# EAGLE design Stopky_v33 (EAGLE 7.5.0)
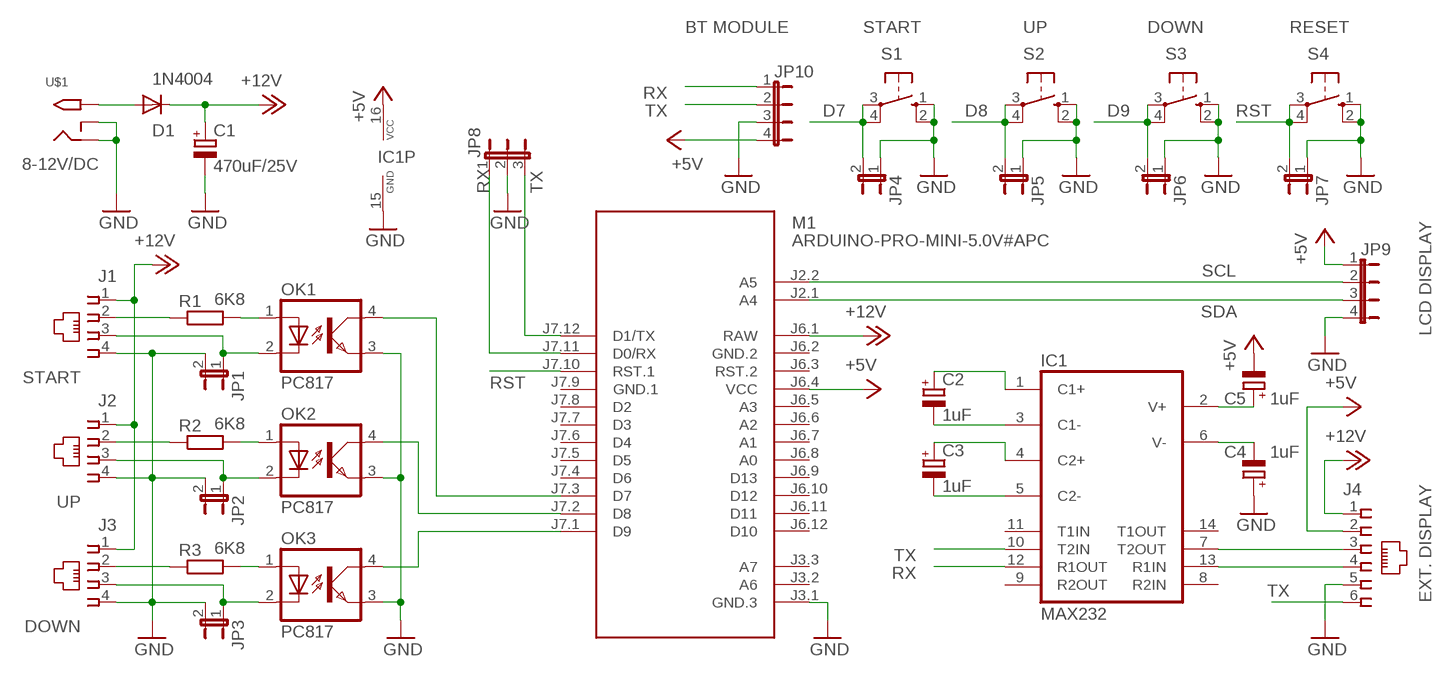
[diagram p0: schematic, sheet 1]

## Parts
C1  470uF/25V  CPOL-EUE3.5-8  [E3,5-8]
C2  1uF  CPOL-EUE2-5  [E2-5]
C3  1uF  CPOL-EUE2-5  [E2-5]
C4  1uF  CPOL-EUE2-5  [E2-5]
C5  1uF  CPOL-EUE2-5  [E2-5]
D1  1N4004  [DO41-10]
IC1  MAX232  [DIL16]
J1  215875-3  [215875-3]
J2  215875-3  [215875-3]
J3  215875-3  [215875-3]
J4  520250-3  [520250-3]
JP1  JP1E  [JP1]
JP2  JP1E  [JP1]
JP3  JP1E  [JP1]
JP4  JP1E  [JP1]
JP5  JP1E  [JP1]
JP6  JP1E  [JP1]
JP7  JP1E  [JP1]
JP8  JP2E  [JP2]
JP9  JP4E  [JP4]
JP10  JP4E  [JP4]
M1  ARDUINO-PRO-MINI-5.0V#APC  [ARDUINO-PRO-MINI#APC]
OK1  PC817  [DIL04]
OK2  PC817  [DIL04]
OK3  PC817  [DIL04]
R1  6K8  R-EU_0207/10  [0207/10]
R2  6K8  R-EU_0207/10  [0207/10]
R3  6K8  R-EU_0207/10  [0207/10]
S1  10-XX  [B3F-10XX]
S2  10-XX  [B3F-10XX]
S3  10-XX  [B3F-10XX]
S4  10-XX  [B3F-10XX]
U$1  2.1MMJACKTHM  [PJ-102A]

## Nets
+5V: C5.- IC1.16(VCC) J4.2 JP9.1 JP10.4 M1.J6.4(VCC)
+12V: C1.+ D1.C J1.1 J2.1 J3.1 J4.1 M1.J6.1(RAW)
D7: JP4.2 M1.J7.3(D7) OK1.4(COL) S1.3(P) S1.4(P1)
D8: JP5.2 M1.J7.2(D8) OK2.4(COL) S2.3(P) S2.4(P1)
D9: JP6.2 M1.J7.1(D9) OK3.4(COL) S3.3(P) S3.4(P1)
GND: C1.- C4.+ IC1.15(GND) J1.4 J2.4 J3.4 J4.5 JP1.2 JP2.2 JP3.2 JP4.1 JP5.1 JP6.1 JP7.1 JP8.2 JP9.4 JP10.3 M1.J3.1(GND.3) OK1.3(EMIT) OK2.3(EMIT) OK3.3(EMIT) S1.1(S) S1.2(S1) S2.1(S) S2.2(S1) S3.1(S) S3.2(S1) S4.1(S) S4.2(S1) U$1.RING U$1.RING_SW
N$1: D1.A U$1.TIP
N$2: J3.2 R3.1
N$3: J2.2 R2.1
N$4: J1.2 R1.1
N$5: OK1.1(A) R1.2
N$6: OK2.1(A) R2.2
N$7: OK3.1(A) R3.2
N$8: C2.+ IC1.1(C1+)
N$9: J1.3 JP1.1 OK1.2(C)
N$10: J2.3 JP2.1 OK2.2(C)
N$11: J3.3 JP3.1 OK3.2(C)
N$15: C2.- IC1.3(C1-)
N$16: C3.+ IC1.4(C2+)
N$17: C3.- IC1.5(C2-)
N$18: C4.- IC1.6(V-)
N$19: C5.+ IC1.2(V+)
N$20: IC1.7(T2OUT) J4.3
N$21: IC1.13(R1IN) J4.4
RST: JP7.2 M1.J7.10(RST.1) S4.3(P) S4.4(P1)
RX: IC1.12(R1OUT) JP8.1 JP10.1 M1.J7.11(D0/RX)
SCL: JP9.2 M1.J2.2(A5)
SDA: JP9.3 M1.J2.1(A4)
TX: IC1.10(T2IN) J4.6 JP8.3 JP10.2 M1.J7.12(D1/TX)
Unconnected: IC1.8(R2IN) IC1.9(R2OUT) IC1.11(T1IN) IC1.14(T1OUT) M1.J3.2(A6) M1.J3.3(A7) M1.J6.3(RST.2) M1.J6.5(A3) M1.J6.6(A2) M1.J6.7(A1) M1.J6.8(A0) M1.J6.9(D13) M1.J6.10(D12) M1.J6.11(D11) M1.J6.12(D10) M1.J7.4(D6) M1.J7.5(D5) M1.J7.6(D4) M1.J7.7(D3) M1.J7.8(D2)

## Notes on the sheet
- BT MODULE | START | UP | DOWN | RESET
- RX
- TX | D7 | D8 | D9 | RST
- 8-12V/DC
- RX | TX
- SCL
- SDA
- LCD DISPLAY
- START
- RST
- UP
- TX
- RX
- TX
- EXT. DISPLAY
- DOWN

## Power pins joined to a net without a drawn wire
GND.1: M1.J7.9(GND.1)
GND.2: M1.J6.2(GND.2)

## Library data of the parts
C1-C5 = rcl:CPOL-EU: POLARIZED CAPACITOR, European symbol
D1 = diode:1N4004: DIODE
IC1 = maxim:MAX232: RS232 TRANSCEIVER; MF: MAXIM; MPN: MAX232ACPE+; OC_FARNELL: 9723773; OC_NEWARK: 68K4544
J1-J3 = con-amp:215875-3: AMP connector
J4 = con-amp:520250-3: AMP connector
JP1-JP7 = jumper:JP1E: JUMPER
JP8 = jumper:JP2E: JUMPER
JP9 JP10 = jumper:JP4E: JUMPER
M1 = Arduino-module:ARDUINO-PRO-MINI-*#APC: Arduino Pro Mini with angle programming connector
OK1-OK3 = optocoupler:PC817: SHARP OPTO COUPLER; MPN: PC817X4J000F; OC_FARNELL: 9707727; OC_NEWARK: 97K7059
R1-R3 = rcl:R-EU_: RESISTOR, European symbol
S1-S4 = switch-omron:10-XX: OMRON SWITCH; MPN: B3F-1000; OC_FARNELL: 176432; OC_NEWARK: 36M3542
U$1 = adafruit:2.1MMJACK: 2.1mm x 5.5mm THM DC jack with internal switch. Digikey part #PJ-102A, 4UCON part #05537 2.1mm x 5.5mm SMT DC jack with internal switch. Digikey part #PJ-002A-SMT, 4UCON part #03267 By microbuilder.eu & adafruit.com

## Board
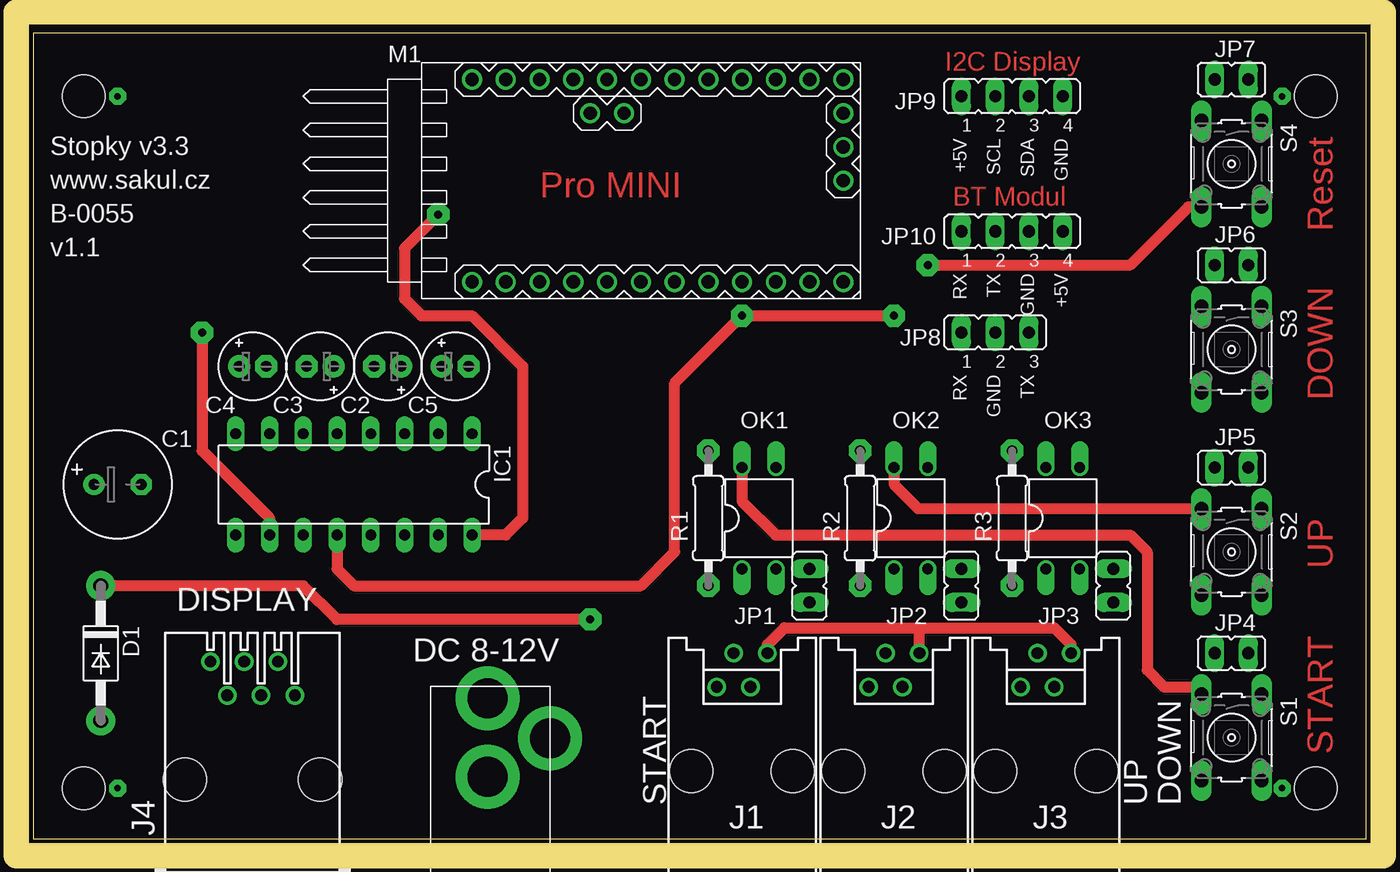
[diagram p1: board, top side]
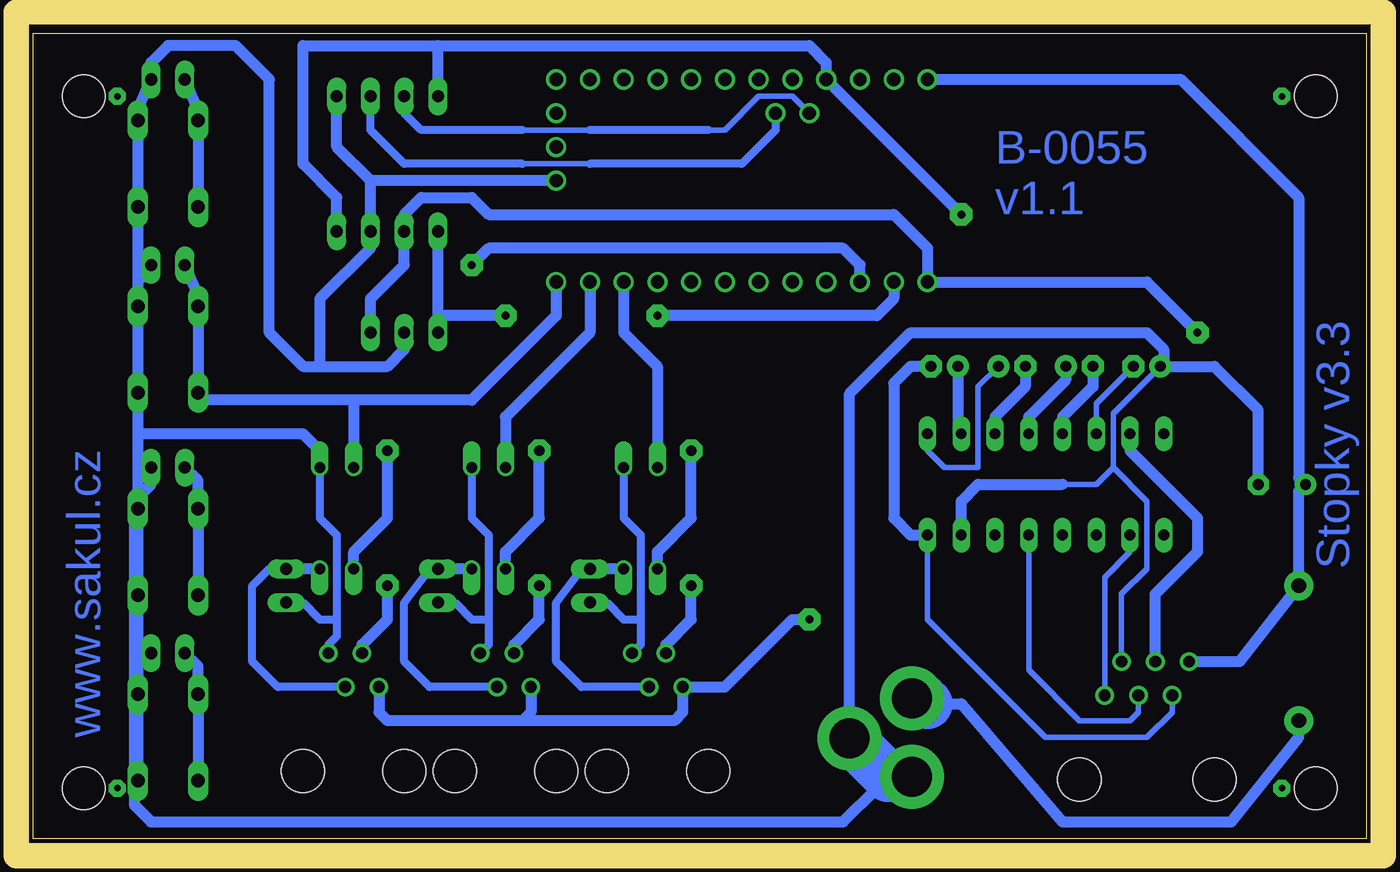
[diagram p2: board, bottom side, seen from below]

Size 100.31 x 60.63 mm. Coordinates in mm from the lower left corner, seen from the top.
Outline: 0,0 100.31,0 100.31,60.63 0,60.63 0,0
Copper layers (1*16): Top 0.035mm / dielectric 1.5mm / Bottom 0.035mm
Design rules "default": minimum track width 10mil, minimum drill 24mil, track to track 8mil, track to pad 8mil, pad to pad 8mil, via to via 8mil, smd to smd 8mil, copper to edge 40mil, drill to drill 8mil, minimum pad ring 10mil, minimum via ring 8mil, stop-mask expansion 4mil, vias tented up to drill 0mil, thermal gap 10mil
Holes 3.2 mm at 3.81,3.81 96.52,3.81 96.52,55.88 3.81,55.88
Milling: 4 lines

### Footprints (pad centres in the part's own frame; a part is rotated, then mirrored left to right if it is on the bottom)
E3,5-8 = drill 0.813 pad 1.6: + -1.778,0 | drill 0.813 pad 1.6 octagon: - 1.778,0
E2-5 = drill 0.813 pad 1.676: + -1.016,0 | drill 0.813 pad 1.676 octagon: - 1.016,0
DO41-10 = drill 1.118 pad 2.184: A 5.08,0; C -5.08,0
DIL16 = drill 0.813 long: 1 -8.89,-3.81; 2 -6.35,-3.81; 3 -3.81,-3.81; 4 -1.27,-3.81; 5 1.27,-3.81; 6 3.81,-3.81; 7 6.35,-3.81; 8 8.89,-3.81; 9 8.89,3.81; 10 6.35,3.81; 11 3.81,3.81; 12 1.27,3.81; 13 -1.27,3.81; 14 -3.81,3.81; 15 -6.35,3.81; 16 -8.89,3.81
215875-3 = drill 0.889: 1 -1.905,6.35; 2 -0.635,8.89; 3 0.635,6.35; 4 1.905,8.89 | hole 3.251: -3.81,0; 3.81,0
520250-3 = drill 0.889: 1 -3.175,8.89; 2 -1.905,6.35; 3 -0.635,8.89; 4 0.635,6.35; 5 1.905,8.89; 6 3.175,6.35 | hole 3.251: -5.08,0; 5.08,0
JP1 = drill 0.914 long: 1 0,-1.27; 2 0,1.27
JP2 = drill 0.914 long: 1 -2.54,0; 2 0,0; 3 2.54,0
JP4 = drill 0.914 long: 1 -3.81,0; 2 -1.27,0; 3 1.27,0; 4 3.81,0
ARDUINO-PRO-MINI#APC = drill 1: J2.1 -1.27,5.08; J2.2 -3.81,5.08; J3.1 15.24,0; J3.2 15.24,2.54; J3.3 15.24,5.08; J6.1 -12.7,7.62; J6.2 -10.16,7.62; J6.3 -7.62,7.62; J6.4 -5.08,7.62; J6.5 -2.54,7.62; J6.6 0,7.62; J6.7 2.54,7.62; J6.8 5.08,7.62; J6.9 7.62,7.62; J6.10 10.16,7.62; J6.11 12.7,7.62; J6.12 15.24,7.62; J7.1 15.24,-7.62; J7.2 12.7,-7.62; J7.3 10.16,-7.62; J7.4 7.62,-7.62; J7.5 5.08,-7.62; J7.6 2.54,-7.62; J7.7 0,-7.62; J7.8 -2.54,-7.62; J7.9 -5.08,-7.62; J7.10 -7.62,-7.62; J7.11 -10.16,-7.62; J7.12 -12.7,-7.62
DIL04 = drill 0.813 offset: 1 -1.27,-3.81; 2 1.27,-3.81; 3 1.27,3.81; 4 -1.27,3.81
0207/10 = drill 0.813 pad 1.676 octagon: 1 -5.08,0; 2 5.08,0
B3F-10XX = drill 1.016 long: 1 -3.251,2.261; 2 3.251,2.261; 3 -3.251,-2.261; 4 3.251,-2.261
PJ-102A = drill 3 pad 4.8: RING 0.1,-3.39; RING_SW -4.6,-6.29; TIP 0.1,-9.29

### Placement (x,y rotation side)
C1  6.35,26.67 0 top
C2  26.67,35.56 180 top
C3  21.59,35.56 180 top
C4  16.51,35.56 0 top
C5  31.75,35.56 0 top
D1  5.08,13.97 270 top
IC1  24.13,26.67 180 top
J1  53.34,5.08 0 top
J2  64.77,5.08 0 top
J3  76.2,5.08 0 top
J4  16.51,4.45 0 top
JP1  58.42,19.05 180 top
JP2  69.85,19.05 180 top
JP3  81.28,19.05 180 top
JP4  90.17,13.97 90 top
JP5  90.17,27.94 90 top
JP6  90.17,43.18 90 top
JP7  90.17,57.15 90 top
JP8  72.39,38.1 0 top
JP9  73.66,55.88 0 top
JP10  73.66,45.72 0 top
M1  45.72,49.53 0 top
OK1  54.61,24.13 0 top
OK2  66.04,24.13 0 top
OK3  77.47,24.13 0 top
R1  50.8,24.13 90 top
R2  62.23,24.13 90 top
R3  73.66,24.13 90 top
S1  90.17,7.62 270 top
S2  90.17,21.59 270 top
S3  90.17,36.83 270 top
S4  90.17,50.8 270 top
U$1  34.29,1.27 180 top

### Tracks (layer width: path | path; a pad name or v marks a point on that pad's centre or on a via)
+5V  (via drill 0.6 pad 1.68)
  Top 0.813: v30.48,46.99 27.94,44.45 27.94,40.64 29.21,39.37 33.02,39.37 36.83,35.56 36.83,24.13 35.56,22.86 IC1.16
  Bottom 0.406: J4.2 14.61,9.53 16.51,7.62 24.13,7.62 33.02,16.51 IC1.16
  Bottom 0.813: JP9.1 69.85,59.69 | 69.85,59.69 41.91,59.69 40.64,58.42 M1.J6.4 v30.48,46.99 | JP10.4 77.47,48.26 80.01,50.8 80.01,59.69 69.85,59.69 | C5.- 34.29,35.56 35.56,34.29 35.56,24.13 34.29,22.86 IC1.16
+12V  (via drill 0.6 pad 1.68)
  Top 0.813: v41.91,16.51 22.86,16.51 20.32,19.05 D1.C
  Bottom 0.813: J4.1 9.53,13.34 D1.C 5.08,26.16 C1.+ 5.08,27.18 5.08,48.26 13.97,57.15 M1.J6.1 | 63.5,8.89 52.07,8.89 51.44,9.53 J1.1 48.26,11.43 43.18,16.51 v41.91,16.51 | 63.5,8.89 73.66,8.89 74.3,9.53 J3.1 | J2.1 62.87,9.53 63.5,8.89
D7
  Top 0.813: OK1.4 53.34,25.4 55.88,22.86 82.55,22.86 83.82,21.59 83.82,12.7 85.09,11.43 87.63,11.43 | 87.63,11.43 87.91,11.43 S1.3 | 87.91,10.16 S1.3 | S1.3 87.91,11.15 87.63,11.43
  Bottom 0.813: JP4.2 87.91,12.98 S1.3 S1.4 | M1.J7.3 55.88,38.1 53.34,35.56 OK1.4
D8
  Top 0.813: OK2.4 64.77,26.67 66.6,24.84 S2.3
  Bottom 0.813: JP5.2 87.91,26.95 S2.3 S2.4 | M1.J7.2 58.42,38.1 64.77,31.75 OK2.4
D9
  Bottom 0.813: JP6.2 87.91,40.92 S3.3 S3.4 87.91,33.02 76.2,33.02 | M1.J7.1 60.96,39.37 67.31,33.02 76.2,33.02 | 76.2,33.02 OK3.4
GND
  Top 0.813: J1.4 55.24,14.61 56.52,15.88 66.67,15.88 | 66.67,15.88 76.83,15.88 78.11,14.61 J3.4 | J2.4 66.67,15.88
  Bottom 0.406: J4.5 18.41,18.41 16.51,20.32 16.51,25.4 19.05,27.94 | 19.05,27.94 19.05,32 C4.+ | 22.86,26.67 20.32,26.67 19.05,27.94
  Bottom 0.61: OK1.3 55.88,24.13 54.61,22.86 54.61,16.51 | 54.61,16.51 54.61,14.61 J1.4 | OK2.3 67.31,24.13 66.04,22.86 66.04,16.51 | 66.04,16.51 66.04,14.61 J2.4 | OK3.3 78.74,24.13 77.47,22.86 77.47,16.51 | 77.47,16.51 77.47,15.24 78.11,14.61 J3.4 | 77.47,16.51 78.74,16.51 80.01,17.78 JP3.2 | JP2.2 68.58,17.78 67.31,16.51 66.04,16.51 | JP1.2 57.15,17.78 55.88,16.51 54.61,16.51
  Bottom 0.813: 92.43,41.91 S4.2 S4.1 92.43,54.89 JP7.1 91.44,58.42 90.17,59.69 85.09,59.69 82.55,57.15 82.55,38.1 80.01,35.56 78.74,35.56 | 92.43,41.91 S3.1 S3.2 92.43,30.48 | 92.43,30.48 92.43,27.94 | 92.43,27.94 S2.1 S2.2 92.43,13.97 | 92.43,13.97 S1.1 S1.2 | JP4.1 92.43,13.97 | 92.43,27.94 JP5.1 91.44,26.67 92.71,25.4 92.71,2.54 91.44,1.27 39.37,1.27 36.83,3.81 | JP6.1 92.43,41.91 | M1.J3.1 74.93,49.53 | 74.93,49.53 77.47,52.07 JP9.4 | 74.93,49.53 JP10.3 74.93,44.45 78.74,40.64 78.74,35.56 | 36.83,3.81 36.83,3.82 35.99,4.66 | OK3.3 78.74,29.21 80.01,30.48 92.43,30.48 | 78.74,35.56 73.66,35.56 72.39,36.83 JP8.2 | C1.- 8.13,32.26 11.43,35.56 C4.+ 15.24,35.81 15.24,36.83 16.51,38.1 34.29,38.1 38.89,33.5 U$1.RING_SW 38.89,5.87 36.83,3.81 | IC1.15 30.48,25.4 29.21,26.67 22.86,26.67
  Bottom 3.81: U$1.RING 35.99,4.66 U$1.RING_SW
N$1
  Bottom 0.813: 33.02,10.16 30.48,10.16 22.86,1.27 10.16,1.27 5.08,7.62 D1.A
  Bottom 3.81: U$1.TIP 33.42,10.56 33.02,10.16
N$2
  Bottom 0.813: J3.2 75.56,14.61 73.66,16.51 R3.1
N$3
  Bottom 0.813: J2.2 64.14,14.61 62.23,16.51 R2.1
N$4
  Bottom 0.813: J1.2 52.7,14.61 50.8,16.51 R1.1
N$5
  Bottom 0.813: OK1.1 53.34,21.59 50.8,24.13 R1.2
N$6
  Bottom 0.813: OK2.1 64.77,21.59 62.23,24.13 R2.2
N$7
  Bottom 0.813: OK3.1 76.2,21.59 73.66,24.13 R3.2
N$8
  Bottom 0.406: IC1.1 33.02,29.21 31.75,27.94 29.21,27.94 29.21,34.04 C2.+
N$9
  Bottom 0.61: J1.3 59.05,11.43 60.96,13.34 60.96,17.78 59.05,20.32 JP1.1
  Bottom 0.813: OK1.2 JP1.1
N$10
  Bottom 0.61: J2.3 70.48,11.43 72.39,13.34 72.39,17.78 70.48,20.32 JP2.1
  Bottom 0.813: OK2.2 JP2.1
N$11
  Bottom 0.61: J3.3 81.92,11.43 83.82,13.34 83.82,19.05 82.55,20.32 JP3.1
  Bottom 0.813: OK3.2 JP3.1
N$15
  Bottom 0.813: C2.- 25.65,34.04 27.94,31.75 IC1.3
N$16
  Bottom 0.813: C3.+ 22.61,34.54 25.4,31.75 IC1.4
N$17
  Bottom 0.813: C3.- 20.57,34.04 22.86,31.75 IC1.5
N$18
  Bottom 0.406: IC1.6 20.32,32.77 C4.-
  Bottom 0.813: 17.78,35.31 C4.-
N$19
  Bottom 0.813: C5.+ 30.73,30.73 IC1.2
N$20
  Bottom 0.813: IC1.7 17.78,29.21 12.7,24.13 12.7,21.59 15.88,18.41 J4.3
N$21
  Bottom 0.406: J4.4 17.14,9.53 17.78,8.89 21.59,8.89 25.4,12.7 IC1.13
N$22  (via drill 0.5 pad 1.27)
  other vias: 6.35,55.88
N$23  (via drill 0.5 pad 1.27)
  other vias: 93.98,55.88
N$24  (via drill 0.5 pad 1.27)
  other vias: 93.98,3.81
N$25  (via drill 0.5 pad 1.27)
  other vias: 6.35,3.81
RST  (via drill 0.6 pad 1.68)
  Top 0.813: v67.31,43.18 82.55,43.18 86.92,47.55 S4.4
  Bottom 0.813: JP7.2 87.91,54.89 S4.3 S4.4 | M1.J7.10 38.1,43.18 39.37,44.45 66.04,44.45 v67.31,43.18
RX  (via drill 0.6 pad 1.68)
  Top 0.813: v64.77,39.37 v53.34,39.37 48.26,34.29 48.26,21.59 45.72,19.05 24.13,19.05 22.86,20.32 IC1.12
  Bottom 0.813: JP8.1 69.85,39.37 | 69.85,39.37 JP10.1 | M1.J7.11 35.56,40.64 36.83,39.37 v53.34,39.37 | v64.77,39.37 69.85,39.37
SCL
  Bottom 0.406: M1.J2.2 43.18,55.88 45.72,55.88 48.26,53.34 49.53,53.34 | 58.42,53.34 63.5,53.34
  Bottom 0.61: 49.53,53.34 58.42,53.34 | 63.5,53.34 71.12,53.34 72.39,54.61 JP9.2
SDA
  Bottom 0.406: 58.42,50.8 63.5,50.8
  Bottom 0.61: M1.J2.1 44.45,53.34 46.99,50.8 58.42,50.8 | 63.5,50.8 72.39,50.8 74.93,53.34 JP9.3
TX  (via drill 0.6 pad 1.68)
  Top 0.813: v12.7,38.1 12.7,29.21 17.78,24.13 IC1.10
  Bottom 0.406: J4.6 19.68,19.68 17.78,21.59 IC1.10
  Bottom 0.813: JP8.3 74.93,40.64 72.39,43.18 JP10.2 72.39,46.99 71.12,48.26 67.31,48.26 66.04,46.99 35.56,46.99 33.02,44.45 M1.J7.12 16.51,41.91 v12.7,38.1

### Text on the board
Top: I2C Display | Pro MINI | BT Modul | Reset | DOWN | UP | START
Bottom: B-0055 | v1.1 | Stopky v3.3 | www.sakul.cz
tPlace: +5V | SCL | SDA | GND | Stopky v3.3 | www.sakul.cz | B-0055 | v1.1 | RX | TX | GND | +5V | RX | GND | TX | DISPLAY | DC 8-12V | START | UP | DOWN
